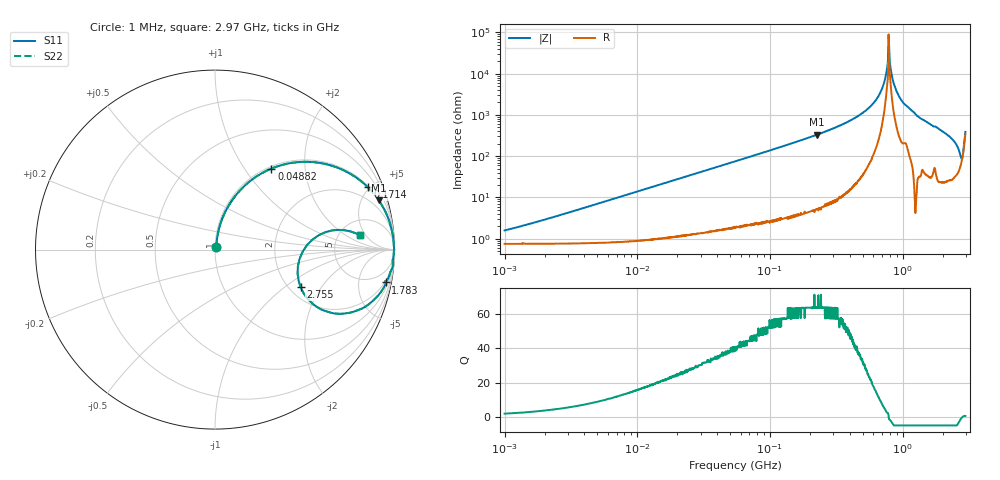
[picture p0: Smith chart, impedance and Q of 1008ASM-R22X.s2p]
!s-Parameter Generated by FASTRON Sdn. Bhd.
!FASTRON P/N : 1008ASM-R22X
!Keysight Technologies: E4991B_MY54100416_A.01.15
!Date: Mon Nov 20 16:16:54 2023
!Version  :Rev00  Wed Nov 22 15:13:35 2023
!Data & Calibration Information:
!Freq  S11  S21  S12  S22
!PortZ  Port1:50+j0  Port2:50+j0
!When reading reference impedance value at option line is always used.
! Remarks : This data is being provided solely for informational purposes.
# Hz S dB R 50
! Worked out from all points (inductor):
!   1599 points, 1 MHz to 2.97 GHz, reference 50 ohm
!   read as one part in series: L = 223 nH near 1.617 MHz
!   highest Q = 63.9 at 225.7 MHz (marker M1), where L = 233 nH
!   self-resonance near 784.7 MHz
!   S11 on the Smith chart (normalised r, x): 1 MHz: 1.02, +0.03; 48.82 MHz: 1.04, +1.34; 171.4 MHz: 1.08, +4.87; 1.783 GHz: 2, -10; 2.755 GHz: 2.29, -1.32; 2.97 GHz: 7.82, +3.63
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1000000  -36.00 61.1  -0.07 -0.8  -0.07 -0.8  -36.00 61.1
3804036  -25.50 78.7  -0.08 -3.0  -0.08 -3.0  -25.50 78.7
1.439846e7  -14.20 76.0  -0.25 -11.2  -0.25 -11.2  -14.20 76.0
4.881767e7  -5.19 55.1  -1.71 -33.3  -1.71 -33.3  -5.19 55.1
5.477226e7  -4.53 52.2  -2.05 -36.4  -2.05 -36.4  -4.53 52.2
1.714156e8  -0.73 22.2  -8.44 -66.8  -8.44 -66.8  -0.73 22.2
2.073156e8  -0.50 18.3  -10.10 -70.8  -10.10 -70.8  -0.50 18.3
2.257233e8  -0.41 16.7  -10.80 -72.4  -10.80 -72.4  -0.41 16.7
3.953438e8  -0.11 8.0  -17.10 -80.8  -17.10 -80.8  -0.11 8.0
5.81181e8  -0.04 3.4  -24.60 -83.9  -24.60 -83.9  -0.04 3.4
7.028992e8  -0.03 1.2  -33.10 -80.7  -33.10 -80.7  -0.03 1.2
7.846996e8  -0.01 0.0  -59.00 -9.4  -59.00 -9.4  -0.01 0.0
8.045804e8  -0.03 -0.3  -44.40 61.5  -44.40 61.5  -0.03 -0.3
8.291033e8  -0.03 -0.6  -39.10 72.5  -39.10 72.5  -0.03 -0.6
8.672962e8  -0.03 -1.1  -34.20 78.7  -34.20 78.7  -0.03 -1.1
9.878038e8  -0.05 -2.6  -26.80 81.8  -26.80 81.8  -0.05 -2.6
1.320433e9  -0.09 -6.3  -19.10 81.7  -19.10 81.7  -0.09 -6.3
1.782824e9  -0.28 -10.9  -14.50 75.1  -14.50 75.1  -0.28 -10.9
2.383164e9  -0.95 -20.8  -8.95 63.0  -8.95 63.0  -0.95 -20.8
2.620866e9  -2.43 -28.1  -6.25 46.9  -6.25 46.9  -2.43 -28.1
2.75535e9  -5.67 -23.7  -4.98 21.8  -4.98 21.8  -5.67 -23.7
2.970126e9  -1.83 5.7  -13.60 -22.4  -13.60 -22.4  -1.83 5.7
